(* Logix 5000 Routine export SetSegStatus; software revision 20.04 *)

TYPE Segment_Status :
STRUCT
   Speed_pulse_status : BOOL; {access Read Only}
   Exists : BOOL; {access Read Only}
   Group_number : INT; {access Read Only}
END_STRUCT
END_TYPE

PROGRAM MainProgram
VAR
   TempStatusPos : INT;
   TempSegStatus : Segment_Status;
   TempGroupNum : INT;
END_VAR

ROUTINE SetSegStatus   (* ladder *)
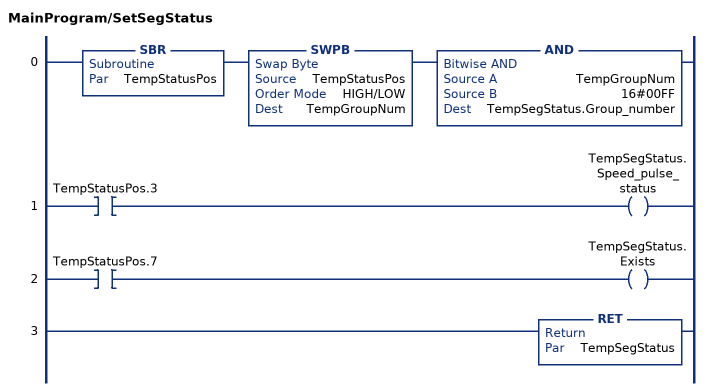
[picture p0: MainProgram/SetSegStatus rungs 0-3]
   0: SBR(TempStatusPos)SWPB(TempStatusPos,HIGH/LOW,TempGroupNum)AND(TempGroupNum,16#00FF,TempSegStatus.Group_number);
   1: XIC(TempStatusPos.3)OTE(TempSegStatus.Speed_pulse_status);
   2: XIC(TempStatusPos.7)OTE(TempSegStatus.Exists);
   3: RET(TempSegStatus);
END_ROUTINE
END_PROGRAM
